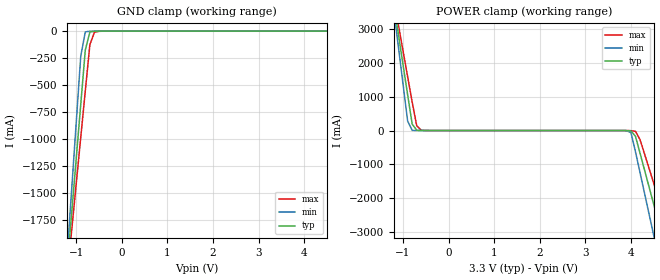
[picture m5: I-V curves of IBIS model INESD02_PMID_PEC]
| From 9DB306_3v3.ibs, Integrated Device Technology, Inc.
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[Model]   INESD02_PMID_PEC
Model_type   Input
Polarity   Non-Inverting
Vinl = 0.8V
Vinh = 2.0V
|   typ   min   max
C_comp   2pF   1.5pF   2.5pF
|   typ   min   max
[Voltage range]  3.3V   3.15V   3.45V
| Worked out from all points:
|   GND clamp passes 1 mA (typ) near -0.54 V on its own axis
|   POWER clamp passes 1 mA (typ) near -0.60 V on its own axis
[GND_clamp]
|Voltage   I(typ)   I(min)   I(max)
-3.3V     -12.83A    -15.14A    -11.37A
-1.2V     -2.195A    -2.092A    -2.281A
-1.1V     -1.689A    -1.472A    -1.849A
-900mV    -678.6mA   -232.7mA   -984.9mA
-800mV    -174mA     -7.255mA   -553.3mA
-700mV    -9.789mA   -1.13mA    -126.1mA
-600mV    -1.72mA    -254.4uA   -11.17mA
-500mV    -427uA     -99.72uA   -2.216mA
6.6V      76.52uA    70.16uA    79.2uA
[POWER_clamp]
|Voltage   I(typ)   I(min)   I(max)
-3.3V     22.38A     26.45A     19.82A
-1.2V     3.723A     3.545A     3.874A
-1.1V     2.836A     2.457A     3.116A
-900mV    1.063A     281mA      1.601A
-800mV    191.6mA    5.071mA    844mA
-600mV    678.1uA    76.63uA    10.7mA
3.9V      -1.629mA   -3.157mA   -831.1uA
4.1V      -173.9mA   -635.2mA   -23.94mA
4.5V      -2.195A    -3.116A    -1.568A
4.7V      -3.206A    -4.358A    -2.433A
4.9V      -4.218A    -5.6A      -3.298A
6.6V      -12.83A    -16.16A    -10.66A
